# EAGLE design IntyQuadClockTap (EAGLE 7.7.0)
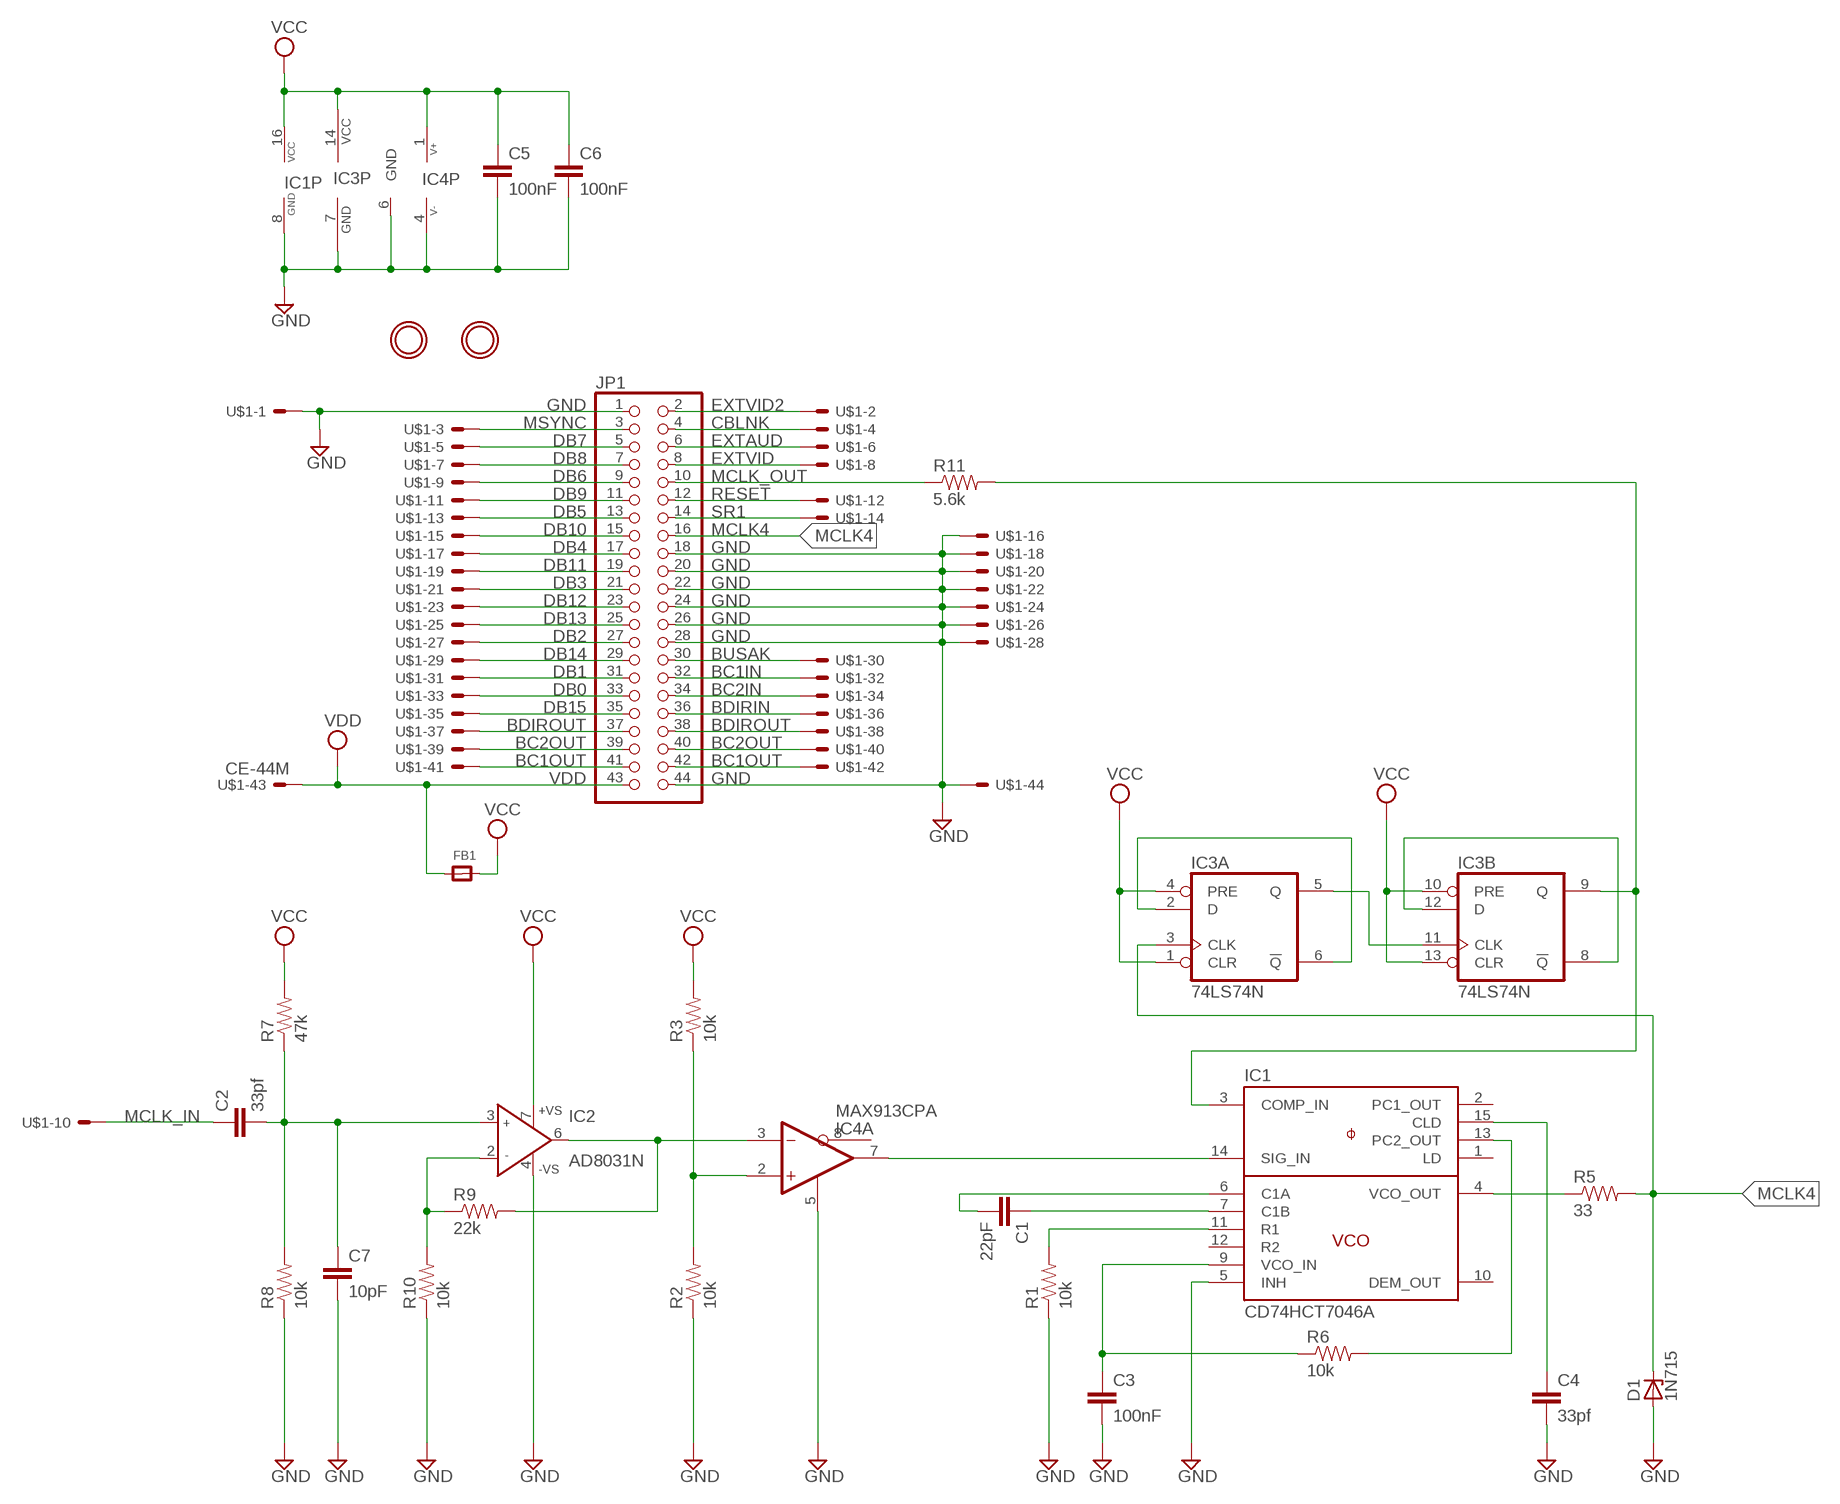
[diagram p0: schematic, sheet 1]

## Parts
C1  22pF  CAPPTH  [CAP-PTH-SMALL]
C2  33pf  CAPPTH  [CAP-PTH-SMALL]
C3  100nF  CAPPTH  [CAP-PTH-SMALL]
C4  33pf  CAPPTH  [CAP-PTH-SMALL]
C5  100nF  CAPPTH  [CAP-PTH-SMALL]
C6  100nF  CAPPTH  [CAP-PTH-SMALL]
C7  10pF  CAPPTH  [CAP-PTH-SMALL]
D1  1N715  ZENER-DIODEZD-10  [ZDIO-10]
FB1  FERRITEPTH_0_6  [FERRITE_0_6]
IC1  CD74HCT7046A  [DIL16]
IC2  AD8031N  [DIL08]
IC3  74LS74N  [DIL14]
IC4  MAX913CPA  [DIL08]
JP1  PINHD-2X22  [2X22]
R1  10k  RESISTORPTH-1/4W  [AXIAL-0.4]
R2  10k  RESISTORPTH-1/4W  [AXIAL-0.4]
R3  10k  RESISTORPTH-1/4W  [AXIAL-0.4]
R5  33  RESISTORPTH-1/4W  [AXIAL-0.4]
R6  10k  RESISTORPTH-1/4W  [AXIAL-0.4]
R7  47k  RESISTORPTH-1/4W  [AXIAL-0.4]
R8  10k  RESISTORPTH-1/4W  [AXIAL-0.4]
R9  22k  RESISTORPTH-1/4W  [AXIAL-0.4]
R10  10k  RESISTORPTH-1/4W  [AXIAL-0.4]
R11  5.6k  RESISTORPTH-1/4W  [AXIAL-0.4]
U$1  CE-44M  [CARDEDGE-44M]
U$2  MOUNTINGHOLE3.0THIN  [MOUNTINGHOLE_3.0_PLATEDTHIN]
U$3  MOUNTINGHOLE3.0THIN  [MOUNTINGHOLE_3.0_PLATEDTHIN]

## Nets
BC1IN: JP1.32 U$1.P$32
BC1OUT: JP1.41 JP1.42 U$1.P$41 U$1.P$42
BC2IN: JP1.34 U$1.P$34
BC2OUT: JP1.39 JP1.40 U$1.P$39 U$1.P$40
BDIRIN: JP1.36 U$1.P$36
BDIROUT: JP1.37 JP1.38 U$1.P$37 U$1.P$38
BUSAK: JP1.30 U$1.P$30
CBLNK: JP1.4 U$1.P$4
DB0: JP1.33 U$1.P$33
DB1: JP1.31 U$1.P$31
DB2: JP1.27 U$1.P$27
DB3: JP1.21 U$1.P$21
DB4: JP1.17 U$1.P$17
DB5: JP1.13 U$1.P$13
DB6: JP1.9 U$1.P$9
DB7: JP1.5 U$1.P$5
DB8: JP1.7 U$1.P$7
DB9: JP1.11 U$1.P$11
DB10: JP1.15 U$1.P$15
DB11: JP1.19 U$1.P$19
DB12: JP1.23 U$1.P$23
DB13: JP1.25 U$1.P$25
DB14: JP1.29 U$1.P$29
DB15: JP1.35 U$1.P$35
EXTAUD: JP1.6 U$1.P$6
EXTVID: JP1.8 U$1.P$8
EXTVID2: JP1.2 U$1.P$2
GND: C3.2 C4.2 C5.2 C6.2 C7.2 D1.A IC1.5(INH) IC1.8(GND) IC2.4(-VS) IC3.7(P:GND) IC4.4(P:V-) IC4.5(A:LE) IC4.6(G:GND) JP1.1 JP1.18 JP1.20 JP1.22 JP1.24 JP1.26 JP1.28 JP1.44 R1.P$1 R2.P$1 R8.P$1 R10.P$1 U$1.P$1 U$1.P$16 U$1.P$18 U$1.P$20 U$1.P$22 U$1.P$24 U$1.P$26 U$1.P$28 U$1.P$44
MCLK4: D1.C IC3.3(A:CLK) JP1.16 R5.P$2
MCLK_IN: C2.1 U$1.P$10
MCLK_OUT: JP1.10 R11.P$1
MSYNC: JP1.3 U$1.P$3
N$1: IC1.11(R1) R1.P$2
N$2: C1.1 IC1.7(C1B)
N$3: C1.2 IC1.6(C1A)
N$4: IC1.14(SIG_IN) IC4.7(A:Q)
N$5: IC2.6(OUT) IC4.3(A:-IN) R9.P$2
N$6: IC4.2(A:+IN) R2.P$2 R3.P$1
N$7: IC3.5(A:Q) IC3.11(B:CLK)
N$8: IC3.2(A:D) IC3.6(A:!Q)
N$9: IC3.8(B:!Q) IC3.12(B:D)
N$10: IC1.3(COMP_IN) IC3.9(B:Q) R11.P$2
N$11: IC1.4(VCO_OUT) R5.P$1
N$13: C4.1 IC1.15(CLD)
N$14: C3.1 IC1.9(VCO_IN) R6.P$1
N$15: IC1.13(PC2_OUT) R6.P$2
N$16: C2.2 C7.1 IC2.3(IN+) R7.P$1 R8.P$2
N$18: IC2.2(IN-) R9.P$1 R10.P$2
RESET: JP1.12 U$1.P$12
SR1: JP1.14 U$1.P$14
VCC: C5.1 C6.1 FB1.P$2 IC1.16(VCC) IC2.7(+VS) IC3.1(A:CLR) IC3.4(A:PRE) IC3.10(B:PRE) IC3.13(B:CLR) IC3.14(P:VCC) IC4.1(P:V+) R3.P$2 R7.P$2
VDD: FB1.P$1 JP1.43 U$1.P$43
Unconnected: IC1.1(LD) IC1.2(PC1_OUT) IC1.10(DEM_OUT) IC1.12(R2) IC4.8(A:!Q)

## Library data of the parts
C1-C7 = SparkFun-Capacitors:CAP: Capacitor
D1 = diode:ZENER-DIODE: Z-Diode
FB1 = microbuilder:FERRITE: Ferrite Bead
IC1 = texas:CD74HCT7046A: Phase-Locked Loop with VCO and Lock Detector
IC2 = analog-devices:AD8031: 2.7 V, 800 ?A, 80 MHz Rail-to-Rail I/O Amplifiers Source: http://www.analog.com/static/imported-files/data_sheets/AD8031_8032.pdf; MPN: AD8031BNZ; OC_FARNELL: 1438575; OC_NEWARK: 15P0920
IC3 = 74xx-us:74*74: Dual D type positive edge triggered FLIP FLOP, preset and clear
IC4 = maxim:MAX913CPA: VOLTAGE COMPARATOR
JP1 = pinhead:PINHD-2X22: PIN HEADER
R1-R3 R5-R11 = SparkFun-Resistors:RESISTOR: Resistor
U$1 = con-cardedge:CE-44M
U$2 U$3 = microbuilder:MOUNTINGHOLE: Mounting Hole

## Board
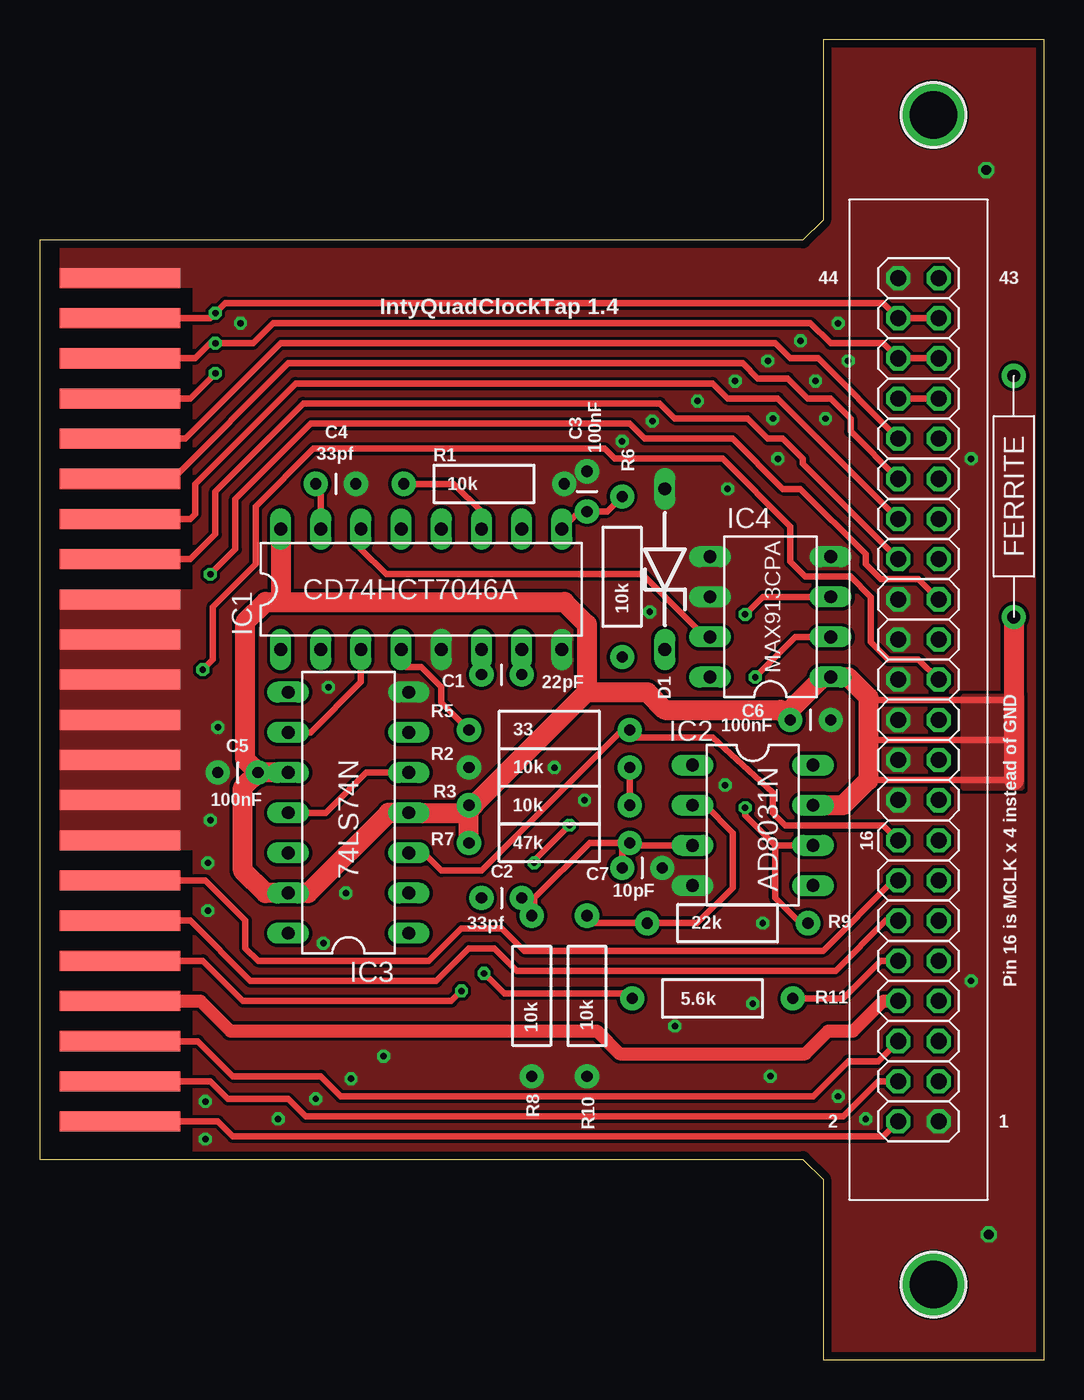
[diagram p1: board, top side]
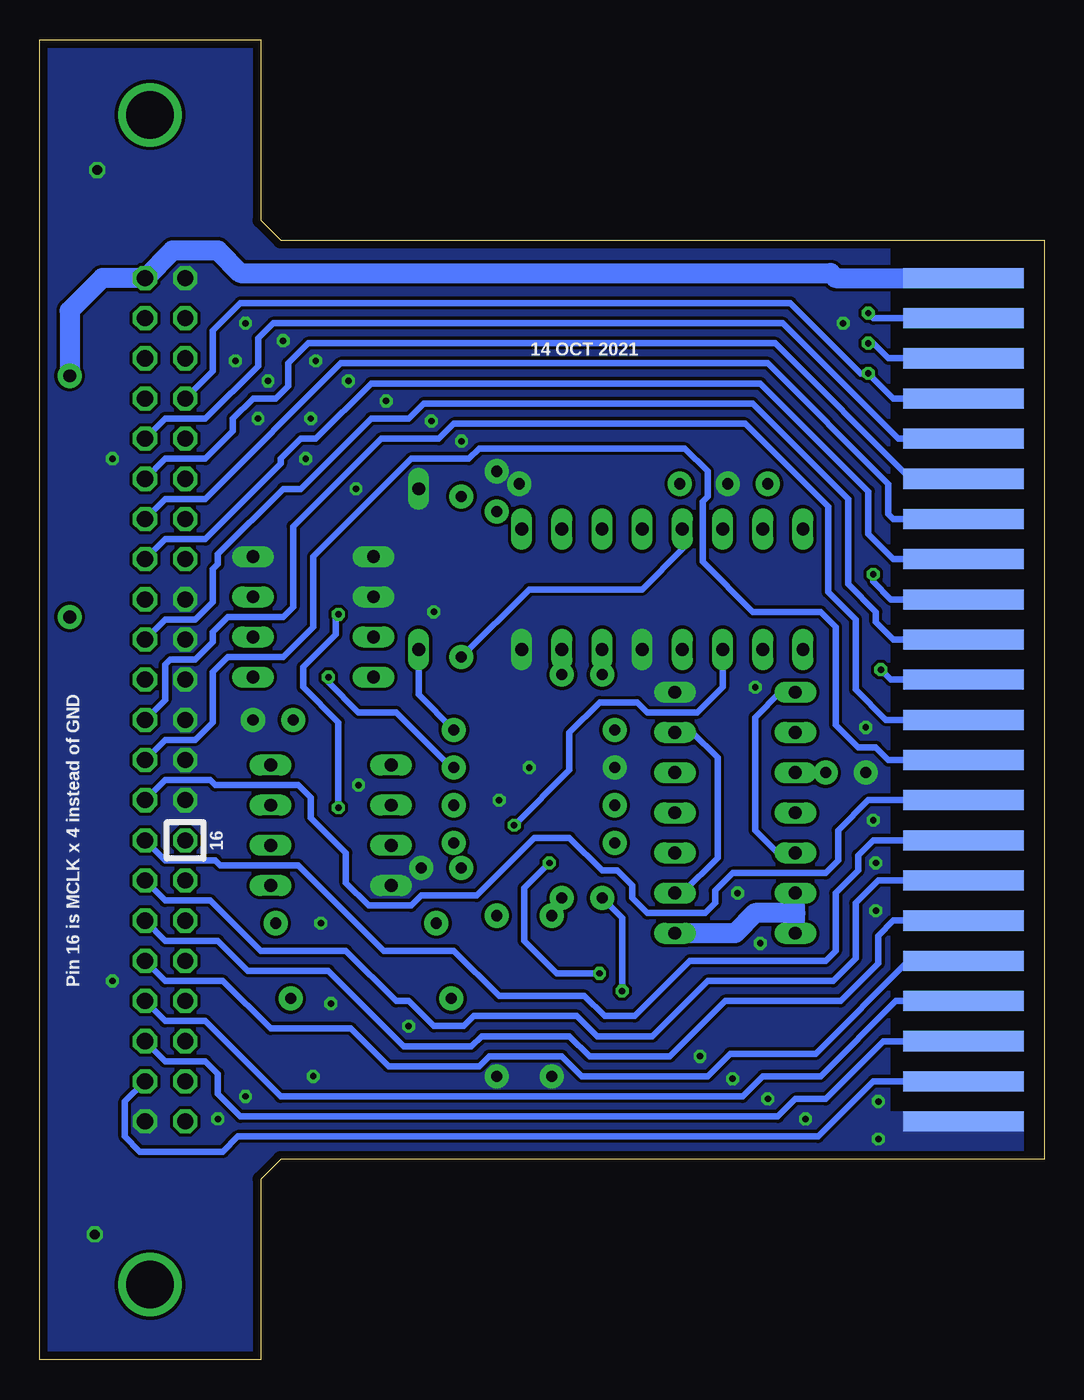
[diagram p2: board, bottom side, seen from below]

Size 63.5 x 83.5 mm. Coordinates in mm from the lower left corner, seen from the top.
Outline: 0,12.7 48.26,12.7 49.53,11.43 49.53,0 63.5,0 63.5,83.5 49.53,83.5 49.53,72.07 48.26,70.8 0,70.8 0,12.7
Copper layers (1*16): Top 0.035mm / dielectric 1.5mm / Bottom 0.035mm
Design rules "default *": minimum track width 10mil, minimum drill 24mil, track to track 8mil, track to pad 8mil, pad to pad 8mil, via to via 8mil, smd to smd 8mil, copper to edge 20mil, drill to drill 8mil, minimum pad ring 10mil, minimum via ring 8mil, stop-mask expansion 4mil, vias tented up to drill 0mil, thermal gap 10mil

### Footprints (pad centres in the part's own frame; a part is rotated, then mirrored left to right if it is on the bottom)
CAP-PTH-SMALL = drill 0.7 pad 1.524: 1 0,0; 2 2.54,0
ZDIO-10 = drill 0.813 long: A 5.08,0; C -5.08,0
FERRITE_0_6 = drill 0.813 pad 1.524: P$1 -7.62,0; P$2 7.62,0
DIL16 = drill 0.813 long: 1 -8.89,-3.81; 2 -6.35,-3.81; 3 -3.81,-3.81; 4 -1.27,-3.81; 5 1.27,-3.81; 6 3.81,-3.81; 7 6.35,-3.81; 8 8.89,-3.81; 9 8.89,3.81; 10 6.35,3.81; 11 3.81,3.81; 12 1.27,3.81; 13 -1.27,3.81; 14 -3.81,3.81; 15 -6.35,3.81; 16 -8.89,3.81
DIL08 = drill 0.813 long: 1 -3.81,-3.81; 2 -1.27,-3.81; 3 1.27,-3.81; 4 3.81,-3.81; 5 3.81,3.81; 6 1.27,3.81; 7 -1.27,3.81; 8 -3.81,3.81
DIL14 = drill 0.813 long: 1 -7.62,-3.81; 2 -5.08,-3.81; 3 -2.54,-3.81; 4 0,-3.81; 5 2.54,-3.81; 6 5.08,-3.81; 7 7.62,-3.81; 8 7.62,3.81; 9 5.08,3.81; 10 2.54,3.81; 11 0,3.81; 12 -2.54,3.81; 13 -5.08,3.81; 14 -7.62,3.81
2X22 = drill 1.016 octagon: 1 -25.4,-1.27; 2 -25.4,1.27; 3 -22.86,-1.27; 4 -22.86,1.27; 5 -20.32,-1.27; 6 -20.32,1.27; 7 -17.78,-1.27; 8 -17.78,1.27; 9 -15.24,-1.27; 10 -15.24,1.27; 11 -12.7,-1.27; 12 -12.7,1.27; 13 -10.16,-1.27; 14 -10.16,1.27; 15 -7.62,-1.27; 16 -7.62,1.27; 17 -5.08,-1.27; 18 -5.08,1.27; 19 -2.54,-1.27; 20 -2.54,1.27; 21 0,-1.27; 22 0,1.27; 23 2.54,-1.27; 24 2.54,1.27; 25 5.08,-1.27; 26 5.08,1.27; 27 7.62,-1.27; 28 7.62,1.27; 29 10.16,-1.27; 30 10.16,1.27; 31 12.7,-1.27; 32 12.7,1.27; 33 15.24,-1.27; 34 15.24,1.27; 35 17.78,-1.27; 36 17.78,1.27; 37 20.32,-1.27; 38 20.32,1.27; 39 22.86,-1.27; 40 22.86,1.27; 41 25.4,-1.27; 42 25.4,1.27; 43 27.94,-1.27; 44 27.94,1.27
AXIAL-0.4 = drill 0.7 pad 1.524: P$1 -5.08,0; P$2 5.08,0
CARDEDGE-44M = smd 7.62 x 1.27 bottom: P$1 0,0; P$3 0,2.54; P$5 0,5.08; P$7 0,7.62; P$9 0,10.16; P$11 0,12.7; P$13 0,15.24; P$15 0,17.78; P$17 0,20.32; P$19 0,22.86; P$21 0,25.4; P$23 0,27.94; P$25 0,30.48; P$27 0,33.02; P$29 0,35.56; P$31 0,38.1; P$33 0,40.64; P$35 0,43.18; P$37 0,45.72; P$39 0,48.26; P$41 0,50.8; P$43 0,53.34 | smd 7.62 x 1.27: P$2 0,0; P$4 0,2.54; P$6 0,5.08; P$8 0,7.62; P$10 0,10.16; P$12 0,12.7; P$14 0,15.24; P$16 0,17.78; P$18 0,20.32; P$20 0,22.86; P$22 0,25.4; P$24 0,27.94; P$26 0,30.48; P$28 0,33.02; P$30 0,35.56; P$32 0,38.1; P$34 0,40.64; P$36 0,43.18; P$38 0,45.72; P$40 0,48.26; P$42 0,50.8; P$44 0,53.34
MOUNTINGHOLE_3.0_PLATEDTHIN = drill 3 pad 3.6: P$1 0,0

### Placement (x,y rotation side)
C1  30.48,43.34 180 top
C2  27.94,29.21 0 top
C3  34.61,53.66 90 top
C4  17.46,55.4 0 top
C5  13.81,37.15 180 top
C6  47.47,40.48 0 top
C7  36.83,31.11 0 top
D1  39.53,50.01 90 top
FB1  61.59,54.61 270 top
IC1  24.13,48.74 0 top
IC2  45.09,33.81 270 top
IC3  19.53,34.61 90 top
IC4  46.2,46.99 90 top
JP1  55.56,40.48 90 top
R1  28.1,55.4 180 top
R2  32.23,37.47 0 top
R3  32.23,35.08 180 top
R5  32.23,39.85 0 top
R6  36.83,49.53 270 top
R7  32.23,32.7 180 top
R8  31.11,23.02 90 top
R9  43.5,27.62 0 top
R10  34.61,23.02 90 top
R11  42.55,22.86 180 top
U$1  5.08,15.08 0 top
U$2  56.52,78.74 0 top
U$3  56.52,4.76 0 top

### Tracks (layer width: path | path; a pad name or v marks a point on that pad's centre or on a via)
BC1IN
  Top 0.406: U$1.P$32 9.53,53.18 9.84,53.5 9.84,55.4 16.19,61.75 42.55,61.75 43.5,60.8 46.67,60.8 JP1.32
BC1OUT  (via drill 0.41)
  Top 0.406: U$1.P$42 10.79,65.88 v11.11,66.2 11.75,66.83 53.34,66.83 JP1.42 JP1.41
  Bottom 0.406: U$1.P$42 10.79,65.88 v11.11,66.2
BC2IN
  Top 0.406: U$1.P$34 8.41,55.72 15.72,63.02 44.45,63.02 45.4,62.07 47.31,62.07 48.58,60.8 50.01,60.8 51.28,59.53 51.28,58.74 JP1.34
BC2OUT  (via drill 0.41)
  Top 0.406: U$1.P$40 9.84,63.34 10.79,64.29 v11.11,64.29 13.49,64.29 14.76,65.56 48.74,65.56 50.01,64.29 53.34,64.29 JP1.40 JP1.39
  Bottom 0.406: v11.11,64.29 10.79,64.29 9.84,63.34 U$1.P$40
BDIRIN
  Top 0.406: U$1.P$36 9.21,58.26 15.24,64.29 46.51,64.29 47.47,63.34 49.21,63.34 JP1.36
BDIROUT  (via drill 0.41)
  Top 0.406: U$1.P$38 9.53,60.8 v11.11,62.39 | JP1.38 JP1.37
  Bottom 0.406: U$1.P$38 9.53,60.8 v11.11,62.39 11.59,62.39 16.03,66.83 50.8,66.83 52.55,65.09 52.55,62.55 JP1.38
BUSAK
  Top 0.406: U$1.P$30 9.53,50.64 11.11,52.23 11.11,54.93 16.67,60.48 39.21,60.48 40.16,59.53 44.77,59.53 46.04,58.26 46.99,58.26 48.26,56.99 48.26,56.67 JP1.30
CBLNK
  Top 0.406: U$1.P$4 10.79,17.62 11.91,16.51 15.72,16.51 16.83,15.4 50.8,15.4 53.02,17.62 JP1.4
DB0
  Bottom 0.406: U$1.P$33 8.41,55.72 16.99,64.29 46.51,64.29 47.78,63.02 47.78,61.59 48.58,60.8 50.01,60.8 51.28,59.53 51.28,58.74 53.02,56.99 55.56,56.99 JP1.33
DB1
  Bottom 0.406: U$1.P$31 9.53,53.18 9.84,53.5 9.84,55.4 17.46,63.02 44.45,63.02 53.02,54.45 55.56,54.45 JP1.31
DB2  (via drill 0.41)
  Top 0.406: v10.79,49.69 12.38,51.28 12.38,54.45 17.14,59.21 37.31,59.21 38.26,58.26 43.81,58.26 46.99,55.09 48.1,55.09 52.23,50.96 52.23,50.32 53.18,49.37 55.56,49.37 JP1.27
  Bottom 0.406: U$1.P$27 9.68,48.1 10.79,49.21 v10.79,49.69
DB3
  Bottom 0.406: U$1.P$21 10,40.48 11.91,42.39 11.91,46.83 13.65,48.58 13.65,53.98 18.89,59.21 37.31,59.21 38.26,58.26 41.91,58.26 47.47,52.7 47.47,47.62 48.1,46.99 51.59,46.99 52.55,46.04 52.55,45.4 53.66,44.29 55.24,44.29 55.56,43.97 55.56,41.75 JP1.21
DB4
  Bottom 0.406: U$1.P$17 11.11,35.4 13.02,33.5 13.02,31.59 13.81,30.8 19.68,30.8 20.8,29.69 20.8,28.89 21.43,28.26 25.08,28.26 26.04,29.21 26.04,30 26.99,30.96 27.94,30.96 30,33.02 32.23,33.02 35.88,29.37 39.37,29.37 40.01,28.73 42.7,28.73 44.13,30.16 44.13,32.07 46.35,34.29 46.35,35.56 47.15,36.35 52.39,36.35 52.7,36.67 55.56,36.67 JP1.17
DB5
  Bottom 0.406: U$1.P$13 10.48,30.32 11.91,28.89 11.91,25.4 13.34,23.97 21.27,23.97 24.77,20.48 28.26,20.48 29.53,21.75 36.04,21.75 36.67,21.11 38.58,21.11 40.16,22.7 40.96,22.7 44.13,25.88 49.53,25.88 52.7,29.05 55.56,29.05 JP1.13
DB6
  Bottom 0.406: U$1.P$9 8.57,25.24 14.45,19.37 19.84,19.37 21.27,17.94 29.21,17.94 30.48,19.21 35.08,19.21 35.72,18.57 41.43,18.57 43.81,20.95 48.9,20.95 51.91,23.97 55.56,23.97 JP1.9
DB7
  Bottom 0.406: U$1.P$5 10.16,20.16 13.81,16.51 15.72,16.51 16.83,15.4 50.8,15.4 52.23,16.83 52.23,18.1 53.02,18.89 55.56,18.89 JP1.5
DB8
  Bottom 0.406: U$1.P$7 9.37,22.7 14.13,17.94 17.78,17.94 19.05,16.67 48.26,16.67 53.02,21.43 55.56,21.43 JP1.7
DB9
  Bottom 0.406: U$1.P$11 9.53,27.78 10.48,26.83 10.48,25.08 12.86,22.7 20.16,22.7 23.65,19.21 28.73,19.21 30,20.48 35.56,20.48 36.2,19.84 40.48,19.84 45.24,24.61 50.32,24.61 52.23,26.51 55.56,26.51 JP1.11
DB10
  Bottom 0.406: U$1.P$15 10.79,32.86 11.75,31.91 11.75,30.96 13.18,29.53 13.18,25.88 13.81,25.24 22.38,25.24 25.88,21.75 27.78,21.75 29.05,23.02 34.45,23.02 37.31,25.88 41.75,25.88 47.15,31.27 52.07,31.27 52.39,31.59 55.56,31.59 JP1.15
DB11
  Bottom 0.406: U$1.P$19 9.84,37.94 10.64,38.73 11.75,38.73 13.18,40.16 13.18,46.35 14.13,47.31 18.41,47.31 21.59,50.48 21.59,54.29 21.27,54.61 21.27,56.2 22.7,57.63 35.72,57.63 36.35,56.99 40.01,56.99 46.2,50.8 46.2,46.35 48.1,44.45 51.59,44.45 52.55,43.5 52.55,40.32 53.66,39.21 55.56,39.21 JP1.19
DB12  (via drill 0.41)
  Top 0.406: v10.32,43.66 10.95,44.29 10.95,47.62 13.65,50.32 13.65,53.98 17.3,57.63 35.72,57.63 36.35,56.99 43.18,56.99 47.47,52.7 47.47,50.48 48.42,49.53 51.28,49.53 52.55,48.26 52.55,45.4 53.66,44.29 55.56,44.29 JP1.23
  Bottom 0.406: U$1.P$23 9.68,43.02 v10.32,43.66
DB13
  Bottom 0.406: U$1.P$25 9.53,45.56 10.64,46.67 10.64,47.31 12.38,49.05 12.38,54.45 18.41,60.48 39.21,60.48 40.16,59.53 42.55,59.53 46.99,55.09 48.1,55.09 52.23,50.96 52.23,50.32 52.55,50.01 52.55,47.94 53.66,46.83 55.56,46.83 JP1.25
DB14
  Bottom 0.406: U$1.P$29 9.53,50.64 11.11,52.23 11.11,54.93 17.94,61.75 42.55,61.75 46.04,58.26 46.99,58.26 48.26,56.99 48.26,56.67 53.02,51.91 55.56,51.91 JP1.29
DB15
  Bottom 0.406: U$1.P$35 9.21,58.26 16.51,65.56 48.74,65.56 49.69,64.61 49.69,62.87 53.02,59.53 55.56,59.53 JP1.35
EXTAUD
  Top 0.406: U$1.P$6 10,20.16 12.22,17.94 17.78,17.94 19.05,16.67 48.9,16.67 51.12,18.89 53.02,18.89 JP1.6
EXTVID
  Top 0.813: U$1.P$8 10.16,22.7 12.06,20.8 35.24,20.8 36.67,19.37 48.42,19.37 49.85,20.8 51.44,20.8 53.34,22.7 JP1.8
EXTVID2
  Top 0.406: U$1.P$2 11.27,15.08 12.22,14.13 53.34,14.13 JP1.2
GND  (via drill 0.41, 0.61)
  other vias: 19.37,29.53 52.23,15.24 50.48,16.67 45.09,22.54 40.16,21.11 46.2,17.94 45.72,27.62 10.79,34.13 43.97,61.91 50.48,65.56 11.27,40.01 48.1,64.45 46.04,63.18 41.59,60.64 10.64,31.43 10.48,13.97 10.48,16.35 38.73,59.37 51.12,63.18 49.05,61.91 49.69,59.53 46.35,59.53 46.67,56.99 43.5,55.09 36.83,58.1 15.08,15.24 17.46,16.51 19.68,17.78 21.75,19.21 18.26,42.55 17.94,26.35 34.45,35.4 32.54,37.47 12.7,65.56 59.85,75.25 60.01,7.94 58.9,56.99 58.9,23.97 38.58,47.31 10.64,28.42 43.34,36.35
  pour Top (isolate 0.203, rank 2, no thermals): 1.42,85.09 101.6,85.09 101.6,-10.79 9.84,-10.79 9.84,32.38 1.42,32.38 1.42,48.58 9.84,48.58 9.84,67.94 1.42,67.94
  pour Bottom (isolate 0.203, no thermals): 9.84,86.36 104.14,86.36 104.14,-12.06 1.42,-12.06 1.42,15.56 9.84,15.56
MCLK4
  Top 0.406: JP1.16 53.34,33.81 47.15,33.81 46.35,34.61 46.35,35.88 42.55,39.37 37.78,39.37 R5.P$2 36.83,39.85 27.94,30.96 25.4,30.96 24.29,32.07 IC3.3
  Bottom 0.406: D1.C 39.53,42.07 R5.P$2
MCLK_IN  (via drill 0.41)
  Top 0.406: U$1.P$10 10.32,25.24 12.86,22.7 26.04,22.7 v26.67,23.34
  Bottom 0.406: v26.67,23.34 26.67,27.94 C2.1
MCLK_OUT
  Top 0.406: JP1.10 53.18,25.24 50.8,22.86 R11.P$1
MSYNC
  Bottom 0.406: U$1.P$3 10.79,17.62 14.29,14.13 50.96,14.13 51.91,13.18 57.15,13.18 58.1,14.13 58.1,16.35 JP1.3
N$1
  Top 0.406: IC1.11 27.94,53.66 26.19,55.4 R1.P$2
N$2
  Top 0.406: C1.1 IC1.7
N$3
  Top 0.406: C1.2 IC1.6
N$4
  Top 0.406: IC1.14 20.32,51.28 21.91,49.69 38.1,49.69 42.07,45.72 IC4.7
N$5  (via drill 0.41)
  Top 0.406: R9.P$2 48.1,27.62 46.51,29.21 46.51,32.54 | 46.51,32.54 IC2.6 | IC4.3 45.72,48.26 v44.61,47.15 | v44.61,34.92 44.61,34.45 46.51,32.54
  Bottom 0.406: v44.61,34.92 44.61,40.32 46.83,42.55 46.83,43.81 44.77,45.88 44.77,46.99 v44.61,47.15
N$6  (via drill 0.41)
  Top 0.406: R2.P$2 R3.P$1 | IC4.2 47.78,45.72 v45.24,43.18
  Bottom 0.406: R2.P$2 37.47,37.47 40.96,40.96 43.34,40.96 45.24,42.86 v45.24,43.18
N$7
  Top 0.406: IC3.11 18.1,34.61 20.64,37.15 IC3.5
N$8
  Bottom 0.406: IC3.2 22.86,29.53 20.64,31.75 20.64,38.1 22.23,39.69 IC3.6
N$9
  Bottom 0.406: IC3.12 16.83,32.07 18.26,33.5 18.26,40.64 16.67,42.23 IC3.8
N$10  (via drill 0.41)
  Top 0.406: IC1.3 20.32,42.86 17.14,39.69 IC3.9 | R11.P$2 37.15,23.18 29.37,23.18 v28.1,24.45 | v31.27,31.43 31.27,31.59 v33.5,33.81
  Bottom 0.406: v28.1,24.45 30.8,24.45 32.86,26.51 32.86,29.84 v31.27,31.43 | v33.5,33.81 30,37.31 30,39.69 28.1,41.59 25.72,41.59 25.08,40.96 21.91,40.96 20.32,42.55 IC1.3
N$11
  Top 0.406: R5.P$1 25.4,41.59 25.4,42.55 24.13,43.81 23.18,43.81 22.86,44.13 IC1.4
N$13
  Top 0.406: IC1.15 17.78,55.09 C4.1
N$14
  Top 0.406: IC1.9 34.13,53.66 C3.1 35.88,53.66 R6.P$1
N$15
  Bottom 0.406: IC1.13 22.86,51.28 25.4,48.74 32.54,48.74 R6.P$2
N$16
  Top 0.406: 31.27,29.21 34.77,32.7 36.83,32.7 | 36.83,32.7 R7.P$1 37.47,32.54 IC2.3 | R8.P$2 31.27,28.26 31.27,29.21 | C7.1 36.83,32.7 | C2.2 31.27,29.21
N$18
  Top 0.406: IC2.2 42.07,35.08 43.81,33.34 43.81,29.84 41.59,27.62 R9.P$1 35.08,27.62 R10.P$2
RESET
  Top 0.406: U$1.P$12 9.53,27.78 13.34,23.97 25.08,23.97 27.15,26.04 28.73,26.04 30.16,24.61 50.32,24.61 53.5,27.78 JP1.12
SR1
  Top 0.406: U$1.P$14 10.48,30.32 13.02,27.78 13.02,26.04 13.81,25.24 24.61,25.24 26.67,27.3 29.21,27.3 30.64,25.88 49.53,25.88 53.98,30.32 JP1.14
VCC
  Top 0.406: 52.39,36.67 61.59,36.67 | 52.39,39.21 61.59,39.21 | 52.39,41.75 61.59,41.75
  Top 1.27: 15.24,47.94 14.29,47.94 13.02,46.67 13.02,37.94 C5.1 | 15.24,47.94 33.18,47.94 34.61,46.51 34.61,42.23 | IC3.10 C5.1 | 34.61,42.23 27.46,35.08 R3.P$2 27.15,34.61 | C5.1 12.86,36.2 12.86,30.96 14.29,29.53 IC3.13 16.99,29.53 22.07,34.61 IC3.4 27.15,34.61 | IC1.16 15.24,47.94 | FB1.P$2 61.59,41.75 61.59,39.21 61.59,36.67 | R7.P$2 27.15,34.61 | IC2.7 50.8,35.08 52.39,36.67 52.39,39.21 52.39,41.75 52.39,41.91 51.12,43.18 IC4.1 49.53,43.18 47.47,41.12 C6.1 46.83,41.12 39.53,41.12 38.42,42.23 34.61,42.23
  Bottom 1.27: IC3.14 15.72,28.26 | 15.72,28.26 IC3.13 | 15.72,28.26 18.26,28.26 19.53,26.99 IC3.1
  pour Top (isolate 0.203, no thermals): 58.42,41.91 62.07,41.91 62.07,36.2 58.42,36.2
VDD
  Bottom 1.27: U$1.P$43 13.18,68.42 13.49,68.74 50.8,68.74 52.23,70.17 55.09,70.17 JP1.43 59.53,68.42 61.59,66.36 FB1.P$1

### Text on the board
tPlace: 44 | 43 | IntyQuadClockTap 1.4 | 16 | Pin 16 is MCLK x 4 instead of GND | 2 | 1
bPlace: 14 OCT 2021 | 16 | Pin 16 is MCLK x 4 instead of GND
